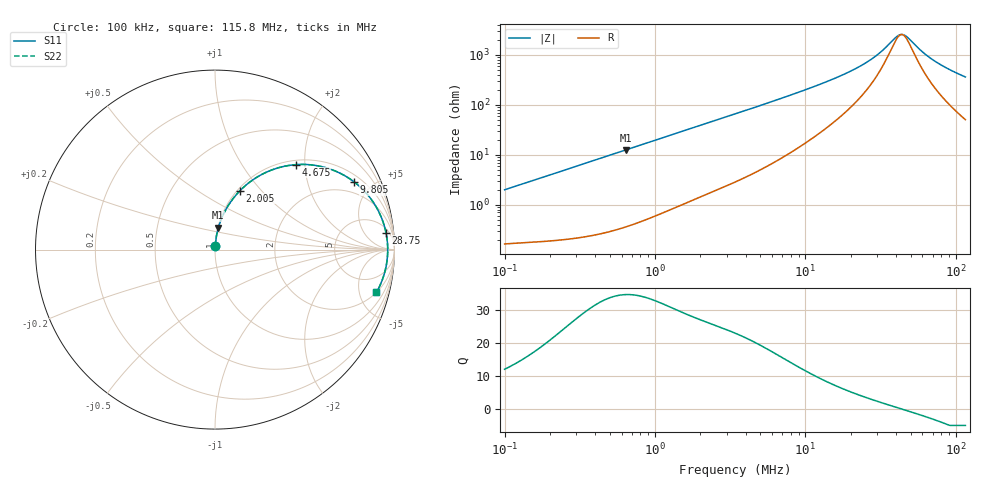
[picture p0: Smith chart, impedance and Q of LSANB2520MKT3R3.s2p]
! LSANB2520MKT3R3  S-PARAMETER MODEL  ( General Type )
! Model Generated by TAIYO YUDEN Corporation (http://www.ty-top.com)
! Version 1.0
! TAIYO YUDEN Control No. 120417NG38SB-FKC
! Copyright(c) 2012 TAIYO YUDEN CO.,LTD. All Rights Reserved.
! Product Description (link to TY-COMPAS)
! https://ds.yuden.co.jp/TYCOMPAS/or/detail?pn=LSANB2520MKT3R3M&u=M
! Products Name : Inductors
! Characteristics :
!  Inductance : 3.3 uH , SRF(min) : -Hz , DC Resistance(max) : 0.156 Ohm
!  Rated Current : Saturation :1800 mA , Temp Rise : 1700 mA (40 degC)
!  Case Size : 2.5 x 2.0 / 0.098 x 0.079 [mm/inch] , Thickness : 1.2 / 0.047 [mm/inch]
!  (Conditions: Temperature = 25 degC , DC Bias Current/Voltage = 0A / 0V)
! External Node Assignments :
!  1  o---GGG---o  2
! GND o---------o GND
! Frequency Range : 0.1MHz  -  115.823372MHz  [ 402 STEP ]
# MHz S RI R 50
! Freq[MHz].  S11 Real  S11 Imag  S21 Real  S21 Imag  S12 Real  S12 Imag  S22 Real  S22 Imag
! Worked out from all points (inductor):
!   401 points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, 100 kHz to 115.8 MHz, reference 50 ohm
!   read as one part in series: L = 3.15 uH near 103.6 kHz
!   highest Q = 34.8 at 637.2 kHz (marker M1), where L = 3.12 uH
!   self-resonance near 43.65 MHz
!   S11 on the Smith chart (normalised r, x): 100 kHz: 1.00, +0.04; 2.005 MHz: 1.03, +0.77; 4.675 MHz: 1.09, +1.80; 9.805 MHz: 1.33, +3.90; 28.75 MHz: 7, +17; 115.8 MHz: 2.01, -7.13
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0.1  0.00203 0.0198  0.998 -0.0198  0.998 -0.0198  0.00203 0.0198
0.325976  0.00628 0.0635  0.9937 -0.0635  0.9937 -0.0635  0.00628 0.0635
0.637157  0.0187 0.122  0.9813 -0.122  0.9813 -0.122  0.0187 0.122
1.062605  0.0467 0.1962  0.9533 -0.1962  0.9533 -0.1962  0.0467 0.1962
2.004995  0.1396 0.3287  0.8604 -0.3287  0.8604 -0.3287  0.1396 0.3287
3.463838  0.3151 0.4433  0.6849 -0.4433  0.6849 -0.4433  0.3151 0.4433
4.674863  0.4506 0.4733  0.5494 -0.4733  0.5494 -0.4733  0.4506 0.4733
6.6521  0.6189 0.4558  0.3811 -0.4558  0.3811 -0.4558  0.6189 0.4558
9.80545  0.774 0.3781  0.226 -0.3781  0.226 -0.3781  0.774 0.3781
11.09389  0.8122 0.3459  0.1878 -0.3459  0.1878 -0.3459  0.8122 0.3459
19.16585  0.9196 0.1962  0.0804 -0.1962  0.0804 -0.1962  0.9196 0.1962
24.10469  0.9417 0.1376  0.0583 -0.1376  0.0583 -0.1376  0.9417 0.1376
28.75388  0.9525 0.0951  0.0475 -0.0951  0.0475 -0.0951  0.9525 0.0951
36.16345  0.9604 0.0422  0.0396 -0.0422  0.0396 -0.0422  0.9604 0.0422
41.64336  0.9622 0.0105  0.0378 -0.0105  0.0378 -0.0105  0.9622 0.0105
43.90604  0.9623 -0.00131  0.0377 0.00131  0.0377 0.00131  0.9623 -0.00131
45.48238  0.9623 -0.0092  0.0377 0.0092  0.0377 0.0092  0.9623 -0.0092
48.80689  0.9617 -0.025  0.0383 0.025  0.0383 0.025  0.9617 -0.025
60.31079  0.9569 -0.0732  0.0431 0.0732  0.0431 0.0732  0.9569 -0.0732
70.68552  0.9496 -0.1106  0.0504 0.1106  0.0504 0.1106  0.9496 -0.1106
90.48224  0.9307 -0.1722  0.0693 0.1722  0.0693 0.1722  0.9307 -0.1722
115.8234  0.8995 -0.2382  0.1005 0.2382  0.1005 0.2382  0.8995 -0.2382
